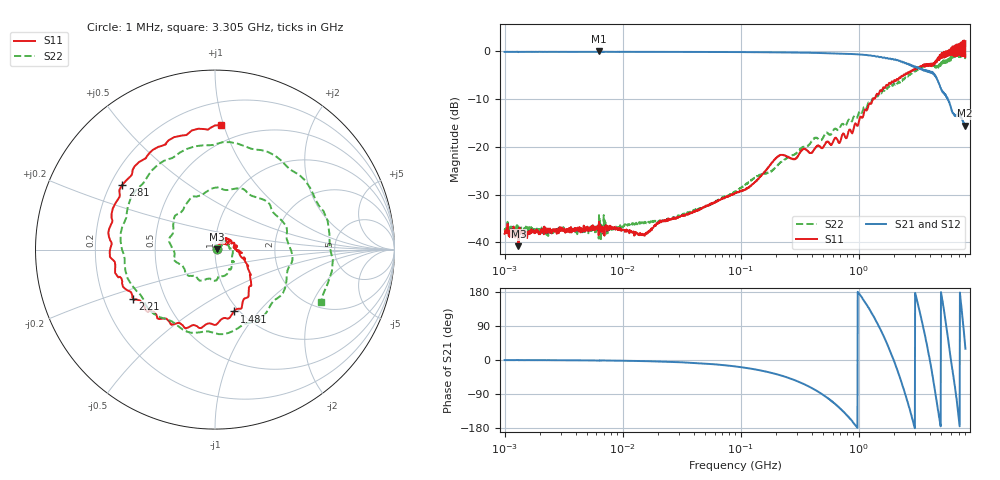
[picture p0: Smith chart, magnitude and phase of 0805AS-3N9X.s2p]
!s-Parameter Generated by FASTRON Sdn. Bhd.
!FASTRON P/N : 0805AS-3N9X
!Keysight Technologies: E5071C_MY46733604_B.14.02
!Date: Mon Jun 15 12:47:02 2026
!Version  :Rev01  Mon Jun 15 12:47:02 2026
!Data & Calibration Information:
!Freq  S11:SOLT2(ON)  S21:SOLT2(ON)  S12:SOLT2(ON)  S22:SOLT2(ON)
!PortZ  Port1:50+j0  Port2:50+j0
!When reading reference impedance value at option line is always used.
! Remarks : This data is being provided solely for informational purposes.
# Hz S dB R 50
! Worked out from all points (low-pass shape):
!   1601 points, 1 MHz to 8 GHz, reference 50 ohm
!   highest |S21| = 0.06 dB at 6.301 MHz (marker M1); lowest = -15.6 dB at 7.923 GHz (marker M2)
!   |S21| within 3 dB of the highest: start of sweep to 2.745 GHz; 2.787 GHz to 2.818 GHz (31.31 MHz wide, 1.12 % of centre)
!   lowest |S11| = -40.8 dB at 1.31 MHz (marker M3), VSWR 1.02, Z = 50.9 + j0.281 ohm
!   |S11| at or under -10 dB: start of sweep to 1.315 GHz
!   |S22| runs from -39.7 to -0.3 dB; largest |S21 - S12| = 0.023
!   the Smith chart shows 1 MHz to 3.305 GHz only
!   S11 on the Smith chart (normalised r, x): 1 MHz: 1.02, +0.00; 1.481 GHz: 0.95, -0.75; 2.21 GHz: 0.33, -0.25; 2.81 GHz: 0.25, +0.30; 3.305 GHz: 0.37, +0.98
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1000000  -38.20 3.5  -0.13 -0.3  -0.11 -0.3  -37.50 3.4
1310238  -40.80 17.6  -0.18 -0.1  -0.14 -0.3  -36.40 -7.1
4479405  -37.40 5.2  -0.13 -0.9  -0.11 -1.0  -37.70 6.2
6301378  -35.70 10.6  0.06 -1.4  -0.10 -0.9  -34.30 18.1
2.00676e7  -35.90 19.9  -0.13 -3.9  -0.14 -3.8  -35.60 24.1
8.994653e7  -29.70 47.4  -0.17 -17.0  -0.17 -17.0  -29.30 34.5
4.006501e8  -21.20 46.8  -0.33 -74.2  -0.33 -74.1  -18.80 -33.6
9.517328e8  -15.30 -15.7  -0.62 -175.0  -0.62 -175.0  -13.90 -147.0
1.481026e9  -8.86 -72.8  -1.20 88.3  -1.18 88.2  -8.88 71.0
1.7949e9  -6.76 -109.0  -1.59 32.3  -1.58 32.1  -7.22 -7.5
2.210346e9  -5.47 -149.0  -1.99 -42.7  -1.99 -43.0  -6.58 -118.0
2.809687e9  -4.01 145.0  -2.90 -150.0  -2.94 -150.0  -4.68 90.9
3.304817e9  -3.17 87.3  -3.56 123.0  -3.58 123.0  -3.61 -26.5
3.852076e9  -2.92 39.7  -4.18 27.1  -4.18 26.9  -2.96 -171.0
4.240668e9  -2.90 -11.1  -4.56 -45.5  -4.54 -45.8  -3.13 98.2
5.052431e9  -0.32 -81.7  -8.13 167.0  -8.14 166.0  -2.24 -130.0
5.64026e9  0.09 -149.0  -9.76 67.1  -9.79 67.0  -1.77 96.4
6.226476e9  1.01 171.0  -12.90 -26.5  -12.90 -27.5  -0.74 -58.3
6.804799e9  0.54 113.0  -13.30 -114.0  -13.40 -114.0  -0.91 -175.0
7.228903e9  1.30 75.7  -13.60 170.0  -13.60 171.0  -0.48 85.8
7.92289e9  1.30 11.1  -15.60 45.7  -15.30 44.8  -0.58 -93.2
8e9  2.10 -7.8  -15.60 29.7  -15.50 29.4  -0.67 -122.0
